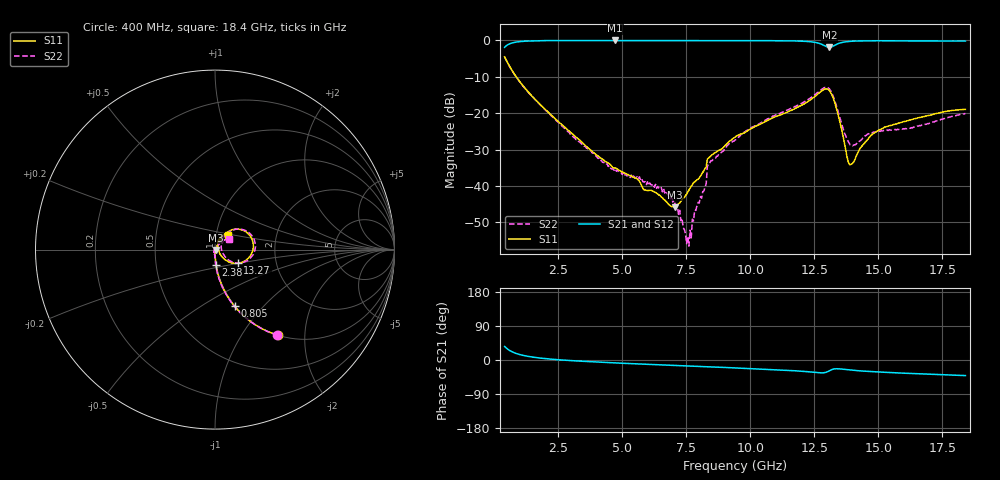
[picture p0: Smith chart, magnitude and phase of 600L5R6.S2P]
!  American Technical Ceramics  Date:  10/27/06
!  One Norden Lane
!  Huntington Station,  NY.  11746-2102
!  Tel:  (631) 622-4700  Fax:  (631) 622-4748
!  Part Number  600L5R6		Mounting Orientation: Vertical
!  Description: Ultra Low ESR Microwave capacitors
!  Application: Coupling, Bypass, Tuning, DC Block
!  Filters, Matching
# GHZ S DB R 50
! Freq  |S11|  S11 Ph  |S21|  S21 Ph  |S12|  S12 Ph  |S22|  S22 Ph
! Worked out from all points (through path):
!   401 points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, 400 MHz to 18.4 GHz, reference 50 ohm
!   highest |S21| = -0.03 dB at 4.72 GHz (marker M1); lowest = -1.9 dB at 13.09 GHz (marker M2)
!   group delay of S21, straight-line fit = 7.87 ps
!   lowest |S11| = -45.8 dB at 7.06 GHz (marker M3), VSWR 1.01, Z = 50.5 - j0.155 ohm
!   |S11| at or under -10 dB: 853 MHz to end of sweep
!   |S22| runs from -56.5 to -4.6 dB; largest |S21 - S12| = 0.0018
!   S11 on the Smith chart (normalised r, x): 400 MHz: 1.00, -1.47; 805 MHz: 1.00, -0.71; 2.38 GHz: 1.00, -0.17; 13.27 GHz: 1.27, -0.20; 18.4 GHz: 1.14, +0.19
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0.4  -4.54 -53.6  -1.92 35.7  -1.91 35.7  -4.60 -54.0
0.805  -9.52 -70.9  -0.53 18.4  -0.53 18.4  -9.59 -71.3
2.38  -21.56 -86.2  -0.05 1.3  -0.04 1.3  -21.71 -87.7
3.415  -27.96 -89.5  -0.04 -3.3  -0.03 -3.3  -28.51 -91.1
4.72  -35.05 -85.7  -0.03 -7.7  -0.03 -7.8  -35.24 -98.5
6.43  -42.52 -64.8  -0.04 -12.7  -0.04 -12.7  -40.58 -117.6
7.06  -45.80 -17.4  -0.04 -14.4  -0.04 -14.5  -45.02 -133.3
7.51  -42.29 22.9  -0.04 -15.7  -0.04 -15.7  -55.86 156.7
7.6  -41.16 28.8  -0.04 -15.9  -0.04 -16.0  -56.55 123.6
7.825  -38.87 34.8  -0.05 -16.5  -0.04 -16.6  -46.66 81.2
8.185  -35.72 49.7  -0.05 -17.6  -0.05 -17.6  -41.38 73.5
8.41  -32.05 62.5  -0.06 -18.2  -0.06 -18.2  -33.78 50.0
9.4  -26.56 62.7  -0.08 -20.8  -0.08 -20.8  -27.38 54.1
12.415  -16.00 45.9  -0.44 -32.0  -0.44 -32.0  -15.54 43.0
12.775  -13.97 28.8  -1.05 -34.0  -1.05 -34.0  -13.51 26.7
13.09  -13.81 -7.5  -1.93 -28.4  -1.93 -28.5  -13.35 -7.3
13.27  -16.57 -30.9  -1.47 -23.6  -1.47 -23.6  -16.01 -28.3
13.675  -28.21 -42.3  -0.45 -24.9  -0.46 -24.9  -25.47 -29.0
13.9  -34.23 6.0  -0.27 -26.5  -0.28 -26.5  -28.75 -4.1
14.71  -26.12 70.0  -0.13 -30.4  -0.13 -30.4  -25.35 42.6
15.43  -23.45 68.0  -0.12 -33.0  -0.12 -33.1  -24.57 44.6
18.4  -18.97 48.3  -0.19 -41.1  -0.19 -41.2  -20.07 36.1
